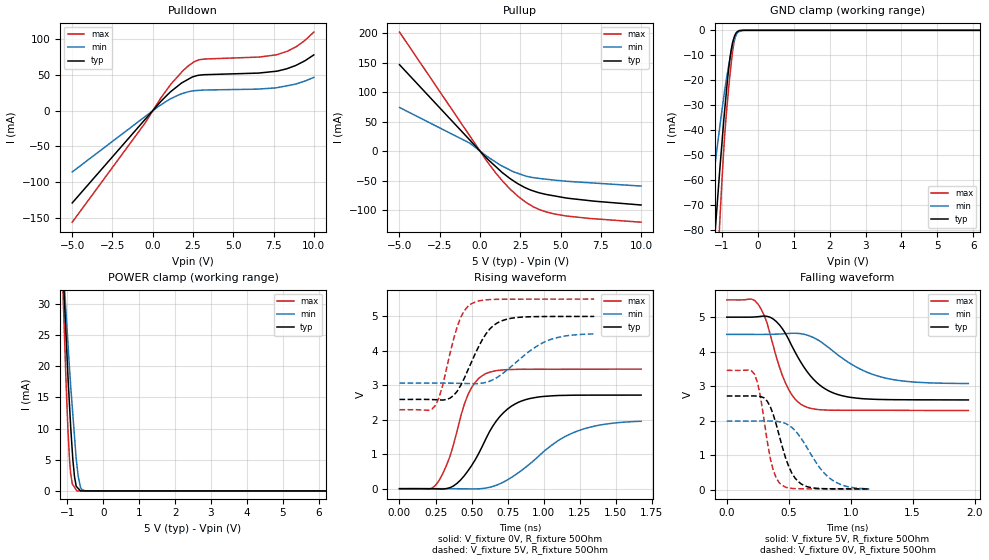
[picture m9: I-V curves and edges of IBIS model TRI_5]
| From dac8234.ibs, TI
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|   tri_5 Model
[Model]   TRI_5
Model_type   3-state
Polarity   Non-Inverting
Enable   Active-Low
Vmeas = 2.5
Vref = 2.5
Cref = 15pF
Rref = 50
|   typ   min   max
|   (nom PVT)   (Fast PVT)   (slow PVT)
|Average
C_comp   3.512e-12   2.849e-12   4.317e-12
|ON state : BUFFER OUTPUT TURNED HIGH
|C_comp   3.797e-12   3.276e-12   4.566e-12
|OFF state: BUFFER in HIGH IMPEDANCE for IOs and 3-state,
|This is BUFFER in LOW state for OUTPUT only type
|C_comp   3.227e-12   2.422e-12   4.067e-12
| Where nom  PVT is Nominal Process, 5V, 42C
|   Fast PVT is Strong Process,  5.5V, -40C
|   Slow PVT is Weak Process,   4.5V, 122C
[Voltage Range]   5   4.5   5.5
|Ambient Temperature   25   105   -40
|Junction Temperature
[Temperature Range]   42   122   -40
[Pullup Reference]   5   4.5   5.5
[Pulldown Reference]   0   0   0
[Power Clamp Reference]   5   4.5   5.5
[GND Clamp Reference]   0   0   0
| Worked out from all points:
|   slope of the pulldown table from 0 to 0.75 V, typ, clamps not added: 40.3 ohm
|   slope of the pullup table from 0 to 0.75 V, typ, clamps not added: 36.4 ohm
|   GND clamp passes 1 mA (typ) near -0.60 V on its own axis
|   POWER clamp passes 1 mA (typ) near -0.76 V on its own axis
|   falling waveform, V_fixture 5V, R_fixture 50Ohm: 20-80 % time 260ps typ, 377ps min, 173ps max; typ from 5 V to 2.6 V
|   rising waveform, V_fixture 0V, R_fixture 50Ohm: 20-80 % time 235ps typ, 374ps min, 154ps max; typ from 0 V to 2.71 V
|   rising waveform, V_fixture 5V, R_fixture 50Ohm: 20-80 % time 171ps typ, 264ps min, 120ps max; typ from 2.59 V to 4.99 V
|   falling waveform, V_fixture 0V, R_fixture 50Ohm: 20-80 % time 140ps typ, 226ps min, 98.1ps max; typ from 2.71 V to 0.018 V
[Pulldown]
|   Voltage   I(typ)   I(min)   I(max)
-5V       -129mA     -85.64mA   -155.9mA
-457mV    -11.67mA   -7.881mA   -16.6mA
500mV     13.01mA    8.146mA    17.8mA
1.138V    27.1mA     17.05mA    37.53mA
1.79V     38.82mA    23.61mA    53.86mA
2.232V    44.37mA    26.68mA    63.19mA
2.574V    47.99mA    28.02mA    68.59mA
3.217V    50.4mA     28.96mA    72.33mA
6.588V    52.69mA    30.36mA    75.04mA
7.766V    55.59mA    32.48mA    78.76mA
8.926V    63.84mA    37.7mA     89.81mA
10V       78.11mA    46.56mA    110mA
[GND Clamp]
|   Voltage   I(typ)   I(min)   I(max)
-5V       -949mA     -662mA     -1.336A
-1.373V   -118.1mA   -76.66mA   -172.2mA
-1.179V   -78.96mA   -52.49mA   -112.3mA
-1.06V    -56.1mA    -38.8mA    -77.1mA
-996mV    -44.73mA   -31.79mA   -59.57mA
-924.5mV  -32.36mA   -24.4mA    -42.65mA
-803.5mV  -14.52mA   -13.58mA   -21.92mA
-740mV    -7.777mA   -8.687mA   -13.12mA
-660.5mV  -2.871mA   -4.083mA   -4.777mA
-594.5mV  -839.4uA   -1.553mA   -1.119mA
-520mV    -102uA     -529.4uA   -212.2uA
10V       0A         0A         0A
[Pullup]
|   Voltage   I(typ)   I(min)   I(max)
-5V       146.5mA    74mA       201.8mA
-617mV    18.24mA    13.22mA    25.04mA
533mV     -15.17mA   -10.72mA   -21.14mA
1.413V    -37.08mA   -25.89mA   -51.34mA
2.37V     -55.65mA   -37.93mA   -76.98mA
2.843V    -62.52mA   -42.35mA   -86.76mA
3.333V    -67.78mA   -45.05mA   -94.79mA
4.163V    -73.78mA   -47.84mA   -103.6mA
4.702V    -76.4mA    -49.46mA   -107mA
6.748V    -83.88mA   -53.62mA   -114.1mA
10V       -91.42mA   -59.29mA   -120.6mA
[POWER Clamp]
|   Voltage   I(typ)   I(min)   I(max)
-5V       299.3mA    258.6mA    355.5mA
-1.123V   35.84mA    36.91mA    32.21mA
-1.081V   30.43mA    32.74mA    25.07mA
-1.034V   24.78mA    28.47mA    17.26mA
-985mV    18.7mA     23.89mA    10.06mA
-935.5mV  13.34mA    19.32mA    4.74mA
-845mV    4.932mA    12.13mA    970.2uA
-800mV    2.265mA    8.705mA    573.7uA
-732mV    612.6uA    4.095mA    0A
-635mV    22.6uA     589.3uA    0A
-486.5mV  0A         0A         0A
10V       0A         0A         0A
[Ramp]
R_load = 50
|   typ   min   max
dV/dt_r   1.6336/2.36311e-10   1.1929/3.86042e-10   2.08208/1.53826e-10
dV/dt_f   1.44734/2.62271e-10   0.862843/3.8351e-10   1.92647/1.73059e-10
[Falling Waveform]
V_fixture = 5V
V_fixture_min = 4.5V
V_fixture_max = 5.5V
R_fixture = 50Ohm
|   Time   V(typ)   V(min)   V(max)
0s        5V         4.5V       5.5V
250ps     5.012V     4.499V     5.389V
325ps     5.024V     4.5V       4.834V
475ps     4.518V     4.521V     3.081V
550ps     3.997V     4.533V     2.63V
625ps     3.54V      4.502V     2.421V
775ps     2.964V     4.246V     2.311V
975ps     2.688V     3.706V     2.298V
1.35ns    2.606V     3.185V     2.297V
1.95ns    2.599V     3.075V     2.292V
[Rising Waveform]
V_fixture = 0V
V_fixture_min = 0V
V_fixture_max = 0V
R_fixture = 50Ohm
|   Time   V(typ)   V(min)   V(max)
0s        1.687nV    2.376nV    1.528nV
250ps     -3.858mV   600.7uV    98.48mV
350ps     28.59mV    57.07uV    938.1mV
475ps     518.7mV    -4.867mV   2.725V
525ps     837.2mV    -7.905mV   3.083V
600ps     1.455V     18.21mV    3.339V
725ps     2.218V     201mV      3.446V
875ps     2.581V     621.9mV    3.462V
1.225ns   2.71V      1.656V     3.462V
1.675ns   2.713V     1.954V     3.466V
[Rising Waveform]
V_fixture = 5V
V_fixture_min = 4.5V
V_fixture_max = 5.5V
R_fixture = 50Ohm
|   Time   V(typ)   V(min)   V(max)
0s        2.587V     3.06V      2.289V
250ps     2.579V     3.061V     2.419V
300ps     2.569V     3.06V      3.004V
400ps     2.824V     3.056V     4.692V
450ps     3.207V     3.05V      5.162V
500ps     3.68V      3.045V     5.364V
600ps     4.491V     3.08V      5.474V
700ps     4.852V     3.289V     5.49V
1.025ns   4.991V     4.29V      5.494V
1.35ns    4.993V     4.486V     5.496V
[Falling Waveform]
V_fixture = 0V
V_fixture_min = 0V
V_fixture_max = 0V
R_fixture = 50Ohm
|   Time   V(typ)   V(min)   V(max)
0s        2.714V     1.987V     3.456V
225ps     2.714V     1.987V     3.339V
275ps     2.694V     1.989V     2.631V
325ps     2.568V     1.99V      1.436V
375ps     2.177V     1.985V     565.1mV
450ps     1.216V     1.947V     113.9mV
525ps     479.2mV    1.803V     34.61mV
625ps     115.5mV    1.351V     21.06mV
850ps     21.59mV    276.5mV    16.2mV
1.15ns    18.2mV     18.91mV    10.87mV
